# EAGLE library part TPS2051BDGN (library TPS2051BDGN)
Single, Current-Limited, Power-Distribution Switch Source: Datasheet
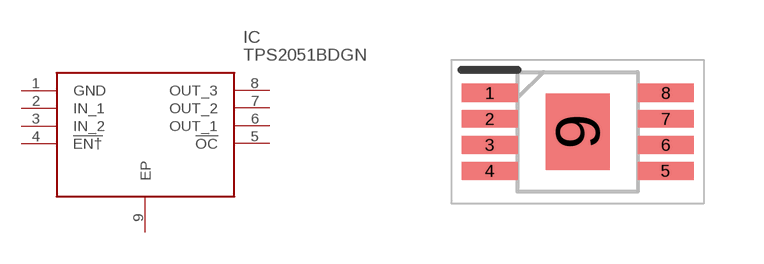
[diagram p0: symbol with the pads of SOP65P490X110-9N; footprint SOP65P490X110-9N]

Designator prefix IC

## TPS2051BDGN (Description: Single, Current-Limited, Power-Distribution Switch; Height: 1.1mm; Manufacturer_Name: Texas Instruments; Manufacturer_Part_Number: TPS2051BDGN; Mouser_Part_Number: 595-TPS2051BDGN; Mouser_Price-Stock: https://www.mouser.co.uk/ProductDetail/Texas-Instruments/TPS2051BDGN?qs=ojKcPFmCWSUKr%252BVWzrslRQ%3D%3D)  [SOP65P490X110-9N]
1  GND
2  IN_1
3  IN_2
4  !EN†
5  !OC
6  OUT_1
7  OUT_2
8  OUT_3
9  EP

## Footprint SOP65P490X110-9N (pad centres in mm)
DGN0008C
smd 1.4 x 0.45: 1 -2.2,0.975; 2 -2.2,0.325; 3 -2.2,-0.325; 4 -2.2,-0.975; 5 2.2,-0.975; 6 2.2,-0.325; 7 2.2,0.325; 8 2.2,0.975
smd 1.6 x 1.92: 9 0,0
